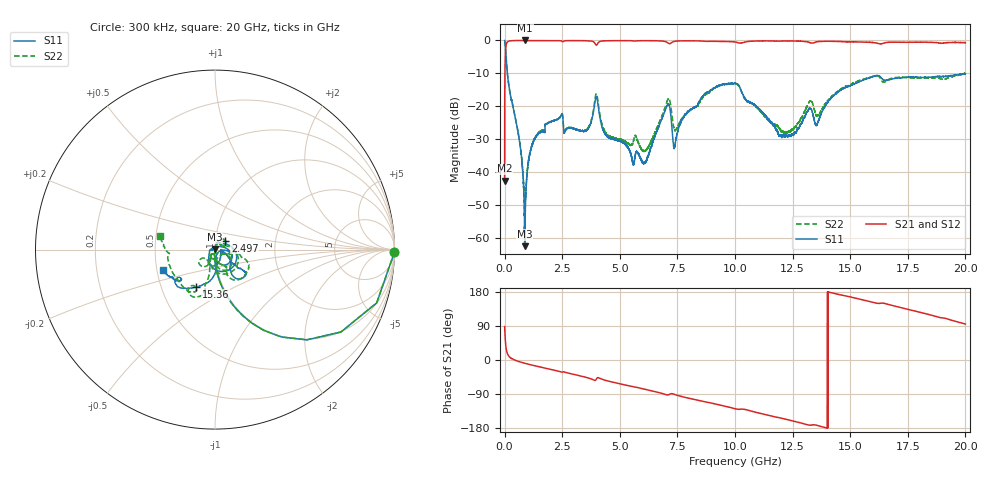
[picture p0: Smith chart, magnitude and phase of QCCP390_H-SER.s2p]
!{QCCP390}
!Johanson Technology Inc.
!www.johansontechnology.com
!Test Board Conditions:
!Substrate Type  RO4350B
!Substrate Thickness  20 mil
!Substrate Dk  3.66
!TL Type: GCPW
!TL Trace Width  36 mil
!TL Gap  12 mil
!Electrode orientation  Horizontal
!DUT TOPOLOGY	SERIES
!Mounting Pad LxW  26x36 mil
! Created Sat Jan  9 18:37:50 2021
# hz S ma R 50
! 2 Port Network Data from SP1.SP block
! freq  magS11  angS11  magS21  angS21  magS12  angS12  magS22  angS22
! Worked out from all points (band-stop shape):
!   20001 points, 300 kHz to 20 GHz, reference 50 ohm
!   highest |S21| = -0.01 dB at 893.3 MHz (marker M1); lowest = -42.6 dB at 300 kHz (marker M2)
!   |S21| within 3 dB of the highest: 40.77 MHz to end of sweep
!   lowest |S11| = -62.5 dB at 880.3 MHz (marker M3), VSWR 1.00, Z = 50 + j0.059 ohm
!   |S11| at or under -10 dB: 119.6 MHz to end of sweep
!   |S22| runs from -52.4 to 0.0 dB; largest |S21 - S12| = 0.017
!   S11 on the Smith chart (normalised r, x): 300 kHz: open; 2.497 GHz: 1.12, +0.11; 15.36 GHz: 0.75, -0.33; 20 GHz: 0.54, -0.14
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300000  0.9997 -0.8  0.007406 88.2  0.007431 89.3  1 -0.8
1.263e8  0.3006 -73.6  0.9516 16.2  0.952 16.1  0.3015 -73.5
6.473e8  0.02927 -95.3  0.9979 -4.6  0.998 -4.6  0.02968 -91.6
8.803e8  0.0007463 127.7  0.9973 -8.6  0.9968 -8.6  0.002806 -0.3
8.933e8  0.001768 112.5  0.9989 -8.8  0.9984 -8.9  0.003088 15.5
1.2963e9  0.03144 78.6  0.9971 -15.0  0.9969 -15.0  0.03213 68.1
2.4973e9  0.07708 40.7  0.9711 -32.3  0.9709 -32.3  0.0771 41.2
3.3343e9  0.04219 51.3  0.9929 -42.7  0.9929 -42.7  0.04237 40.1
3.9863e9  0.1392 -49.9  0.8464 -50.0  0.8464 -49.9  0.1554 -51.3
4.4423e9  0.03495 -151.8  0.9891 -54.7  0.9877 -54.7  0.03774 -124.2
6.0523e9  0.01369 107.9  0.9916 -76.7  0.9932 -76.7  0.02062 -82.7
6.6673e9  0.0468 17.7  0.9882 -85.6  0.9871 -85.5  0.05199 -24.5
7.1003e9  0.1082 -37.9  0.9131 -92.2  0.9134 -92.2  0.1297 -48.0
7.3923e9  0.02542 -24.9  0.9715 -91.2  0.9722 -91.3  0.04267 -58.0
8.6743e9  0.1534 -37.7  0.9735 -110.3  0.9741 -110.3  0.1467 -13.2
1.00003e10  0.2221 -42.6  0.9482 -128.5  0.9475 -128.5  0.218 -43.1
1.20993e10  0.03536 -6.1  0.9812 -154.7  0.984 -154.7  0.04052 -126.9
1.33343e10  0.08655 -115.1  0.9113 -171.6  0.9127 -171.7  0.1175 -139.3
1.36043e10  0.05764 -90.4  0.961 -173.2  0.9613 -173.3  0.07315 -124.3
1.53603e10  0.2333 -116.6  0.9495 161.3  0.9547 161.1  0.2447 -104.4
1.66673e10  0.2519 -138.3  0.939 146.5  0.9297 146.4  0.2546 -114.8
2e10  0.3114 -158.3  0.9272 94.8  0.9179 94.8  0.3194 166.5
